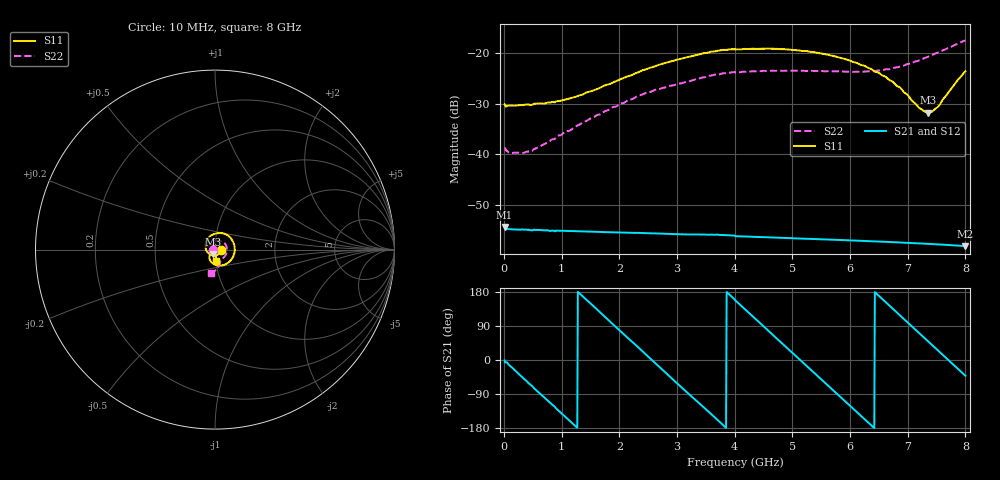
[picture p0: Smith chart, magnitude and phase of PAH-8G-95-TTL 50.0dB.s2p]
! MTS Systemtechnik GmbH
! S-Parameters
! Model: PAH-8G/95-TTL
! Attenuation Step: 50.0dB
! Rohde & Schwarz ZVB8 2Ports - Version 4.11 - 1145.1010k08 SN: 100119
! S2P File Measurements:
! S11 S21 S12 S22
# HZ  S  DB  R  50.00
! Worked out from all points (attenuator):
!   800 points, 10 MHz to 8 GHz, reference 50 ohm
!   highest |S21| = -54.45 dB at 10 MHz (marker M1); lowest = -58.2 dB at 8 GHz (marker M2)
!   lowest |S11| = -31.8 dB at 7.35 GHz (marker M3), VSWR 1.05, Z = 49.1 - j2.38 ohm
!   |S11| at or under -10 dB: start of sweep to end of sweep
!   |S22| runs from -39.8 to -17.5 dB; largest |S21 - S12| = 2.6e-05
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1e7  -30.16 -4.0  -54.45 -1.1  -54.35 -1.1  -38.81 -168.9
1.2e8  -30.38 -11.8  -54.90 -17.7  -54.91 -17.7  -39.80 177.5
4.6e8  -30.29 -44.5  -55.07 -65.4  -55.10 -65.1  -39.48 172.4
9e8  -29.58 -89.5  -55.16 -127.4  -55.18 -127.5  -36.64 164.2
1.35e9  -28.29 -135.5  -55.33 169.9  -55.34 169.9  -33.87 150.5
2.31e9  -23.89 143.2  -55.62 35.9  -55.62 35.9  -28.56 109.5
2.68e9  -22.35 117.3  -55.75 -16.5  -55.75 -16.2  -27.18 93.2
3.44e9  -20.12 68.7  -55.96 -121.7  -55.98 -122.1  -24.86 58.0
4.01e9  -19.30 32.5  -56.26 157.3  -56.26 157.3  -23.87 31.1
4.67e9  -19.15 -7.9  -56.54 65.0  -56.56 65.0  -23.51 1.8
5.34e9  -19.80 -48.9  -56.82 -28.4  -56.83 -28.4  -23.53 -26.0
5.73e9  -20.63 -72.6  -56.98 -82.8  -57.01 -82.8  -23.64 -39.8
6.11e9  -21.92 -95.7  -57.15 -136.3  -57.17 -136.3  -23.70 -50.8
6.36e9  -23.11 -109.8  -57.28 -171.2  -57.28 -171.3  -23.61 -56.5
6.67e9  -25.25 -124.8  -57.42 145.3  -57.43 145.3  -23.22 -62.5
6.87e9  -26.86 -131.1  -57.52 117.1  -57.54 117.1  -22.63 -66.6
7.2e9  -30.86 -124.6  -57.70 70.7  -57.71 70.7  -21.45 -73.5
7.35e9  -31.78 -109.5  -57.79 49.6  -57.80 49.6  -20.73 -76.9
7.42e9  -31.61 -101.6  -57.84 39.8  -57.84 39.7  -20.42 -79.0
7.53e9  -30.61 -90.2  -57.90 24.3  -57.92 24.3  -19.88 -81.9
7.85e9  -25.58 -81.9  -58.11 -20.6  -58.14 -20.7  -18.24 -92.7
8e9  -23.61 -85.1  -58.25 -41.5  -58.25 -41.5  -17.51 -98.5
